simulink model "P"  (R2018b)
settings: Solver=VariableStepAuto  StartTime=0.0  StopTime=10.0  RelTol=1e-3

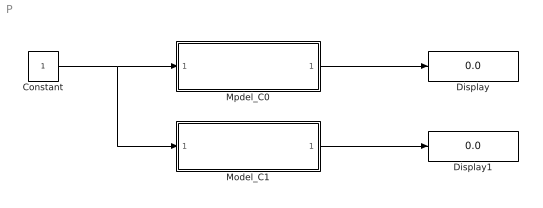
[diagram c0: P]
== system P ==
  Constant : Constant
  Display : Display
  Display1 : Display
  Model_C1 : ModelReference  ModelNameDialog=C1.slx  SimulationMode=Normal  ModelReferenceVersion=1.2
  Mpdel_C0 : ModelReference  ModelNameDialog=C0.slx  SimulationMode=Normal  ModelReferenceVersion=1.2
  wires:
  Mpdel_C0/1 -> Display/1
  Model_C1/1 -> Display1/1
  Constant/1 -> Model_C1/1, Mpdel_C0/1
